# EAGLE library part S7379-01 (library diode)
Si PIN Quadrant photodiode Source: http://sales.hamamatsu.com/assets/pdf/parts_S/S7379-01_etc.pdf
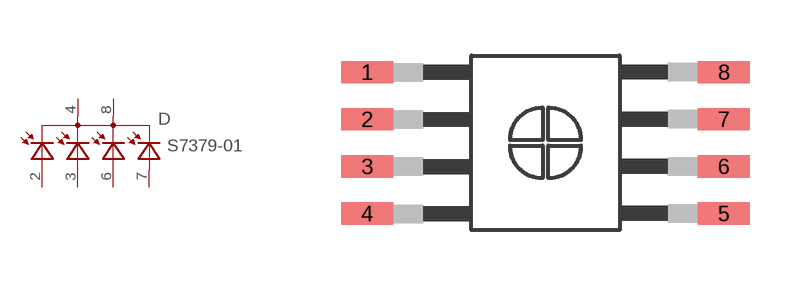
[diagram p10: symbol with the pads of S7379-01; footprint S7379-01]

Designator prefix D

## S7379-01  [S7379-01]
2  AA  pas
3  AB  pas
4  C1  pas
6  AC  pas
7  AD  pas
8  C2  pas

## Footprint S7379-01 (pad centres in mm)
Si PIN Quadrant photodiode Source: http://sales.hamamatsu.com/assets/pdf/parts_S/S7379-01_etc.pdf
smd 1.4 x 0.6: 1 -4.805,1.905; 2 -4.805,0.635; 3 -4.805,-0.635; 4 -4.805,-1.905; 5 4.805,-1.905; 6 4.805,-0.635; 7 4.805,0.635; 8 4.805,1.905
